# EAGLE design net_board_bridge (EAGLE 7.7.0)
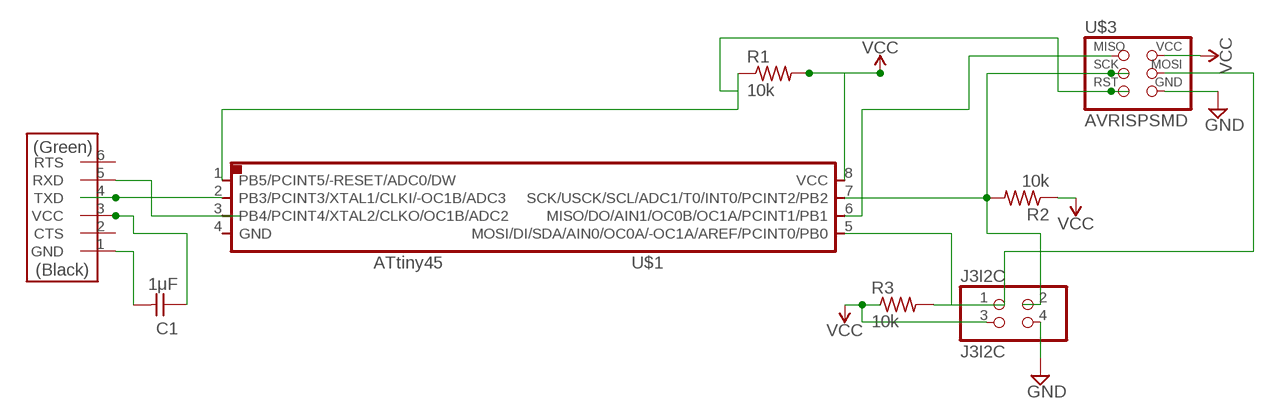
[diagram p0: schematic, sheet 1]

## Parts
C1  1μF  CAP-UNPOLARIZEDFAB  [C1206FAB]
J3I2C  J3I2C  PINHD-2X2-SMD  [2X02SMD]
R1  10k  RES-US1206FAB  [R1206FAB]
R2  10k  RES-US1206FAB  [R1206FAB]
R3  10k  RES-US1206FAB  [R1206FAB]
U$1  ATTINY45SI  [SOIC8]
U$2  FTDI-SMD-HEADER  [1X06SMD]
U$3  AVRISPSMD  [2X03SMD]

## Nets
GND: J3I2C.4 U$3.6(GND)
N$2: R1.1 U$1.1(PB5/PCINT5/-RESET/ADC0/DW) U$3.5(RST)
N$3: U$2.5(RXD)
N$4: R2.2 U$1.7(SCK/USCK/SCL/ADC1/T0/INT0/PCINT2/PB2) U$3.3(SCK)
N$6: R3.2 U$1.5(MOSI/DI/SDA/AIN0/OC0A/-OC1A/AREF/PCINT0/PB0) U$3.4(MOSI)
N$7: U$1.2(PB3/PCINT3/XTAL1/CLKI/-OC1B/ADC3) U$2.4(TXD)
N$8: C1.2 U$2.1(GND)
N$9: C1.1 U$2.3(VCC)
N$11: U$1.6(MISO/DO/AIN1/OC0B/OC1A/PCINT1/PB1) U$3.1(MISO)
VCC: J3I2C.3 R1.2 R2.1 R3.1 U$1.8(VCC) U$3.2(VCC)
Unconnected: J3I2C.1 J3I2C.2 U$1.3(PB4/PCINT4/XTAL2/CLKO/OC1B/ADC2) U$1.4(GND) U$2.2(CTS) U$2.6(RTS)

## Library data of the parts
C1 = fab:CAP-UNPOLARIZED
J3I2C = fab:PINHD-2X2-SMD
R1-R3 = fab:RES-US: Resistor (US Symbol)
U$1 = fab:ATTINY45
U$2 = fab:FTDI-SMD-HEADER
U$3 = fab:AVRISP

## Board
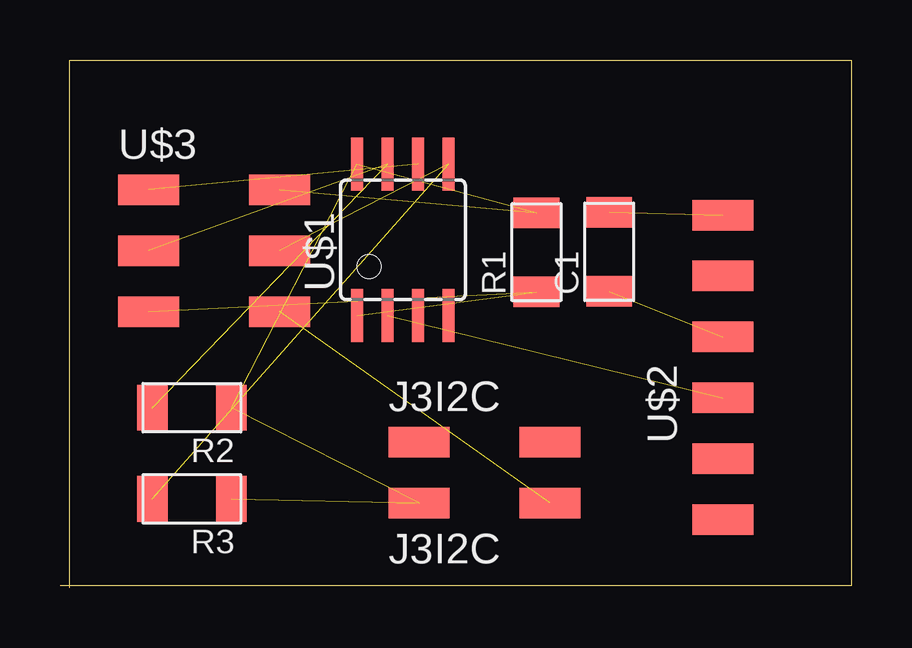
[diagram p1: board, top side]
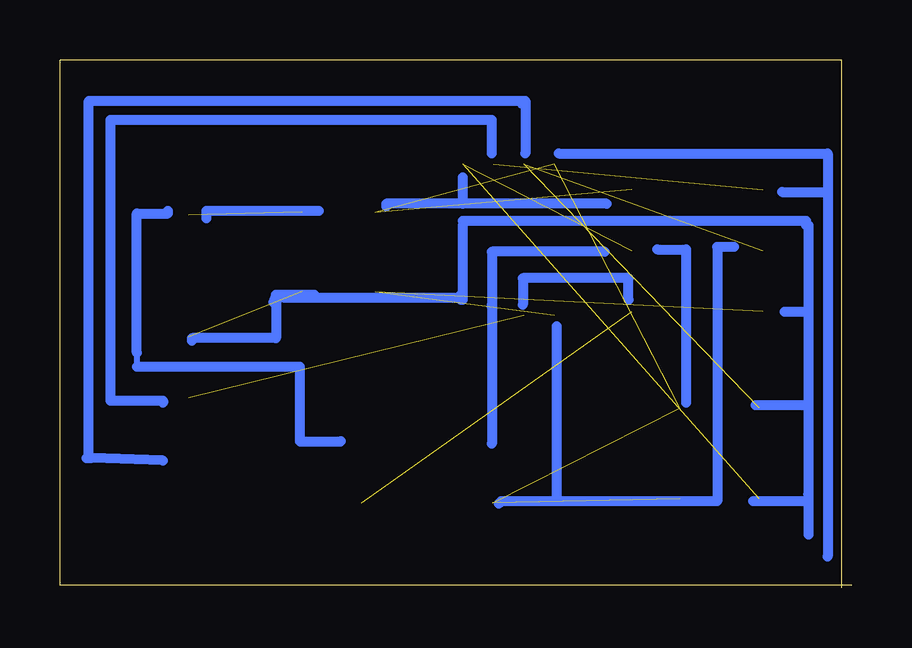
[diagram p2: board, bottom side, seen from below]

Size 33 x 22 mm. Coordinates in mm from the lower left corner, seen from the top.
Outline: 0,0.1 33,0.1 33,22 0.4,22 0.4,0
Copper layers (1*16): Top 0.035mm / dielectric 1.5mm / Bottom 0.035mm
Design rules "default": minimum track width 10mil, minimum drill 24mil, track to track 8mil, track to pad 8mil, pad to pad 8mil, via to via 8mil, smd to smd 8mil, copper to edge 40mil, drill to drill 8mil, minimum pad ring 10mil, minimum via ring 8mil, stop-mask expansion 4mil, vias tented up to drill 0mil, thermal gap 10mil

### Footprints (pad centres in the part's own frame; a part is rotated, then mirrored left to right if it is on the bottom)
C1206FAB = smd 1.27 x 1.905: 1 -1.651,0; 2 1.651,0
2X02SMD = smd 2.54 x 1.27: 1 -2.54,1.27; 2 2.92,1.27; 3 -2.54,-1.27; 4 2.92,-1.27
R1206FAB = smd 1.27 x 1.905: 1 -1.651,0; 2 1.651,0
SOIC8 = smd 0.5 x 2.2: 1 -1.905,-3.154; 2 -0.645,-3.154; 3 0.625,-3.154; 4 1.895,-3.154; 5 1.905,3.154; 6 0.635,3.154; 7 -0.635,3.154; 8 -1.905,3.154
1X06SMD = smd 2.54 x 1.27: 1 0,6.35; 2 0,3.81; 3 0,1.27; 4 0,-1.27; 5 0,-3.81; 6 0,-6.35
2X03SMD = smd 2.54 x 1.27: 1 -2.54,2.54; 2 2.92,2.54; 3 -2.54,0; 4 2.92,0; 5 -2.54,-2.54; 6 2.92,-2.54

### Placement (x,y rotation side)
C1  22.9,14 90 top
J3I2C  17.5,4.8 0 top
R1  19.86,13.98 90 top
R2  5.5,7.5 180 top
R3  5.5,3.7 180 top
U$1  14.3,14.5 0 top
U$2  27.64,9.18 0 top
U$3  6.23,14.05 0 top

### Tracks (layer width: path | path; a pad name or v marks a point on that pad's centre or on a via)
GND  (1 unrouted)
N$1
  Bottom 0.406: 22.2,15.7 26.9,15.7 26.9,15.4
N$2  (2 unrouted)
N$4  (2 unrouted)
N$5
  Bottom 0.406: 22.4,12.2 24,12.2 | 24.1,11.9 24,12.2 | 24,12.2 24,10.4 27.5,10.4 27.5,10.3
N$6  (2 unrouted)
N$7  (1 unrouted)
N$8  (1 unrouted)
N$9  (1 unrouted)
N$10
  Bottom 0.406: 23.7,12.1 16.3,12.1 16.3,12.2
N$11  (1 unrouted)
N$12
  Bottom 0.406: 7.5,3.6 12.3,3.6 | 12.3,3.6 14.6,3.6 14.7,3.5 | 12.3,10.9 12.3,3.6
N$13
  Bottom 0.406: 10.3,14 15,14 15,11.8 | 15,11.8 15,11.7 | 15,11.8 15,6
N$14
  Bottom 0.406: 16.3,12 16.2,12 16.2,15.1
N$15
  Bottom 0.406: 16.2,15.3 1.9,15.3
N$16
  Bottom 0.406: 2,3.6 4.1,3.6
N$17
  Bottom 0.406: 1.9,7.6 4,7.6
N$18
  Bottom 0.406: 1.9,15.1 1.8,15.1 1.8,3.7
N$19
  Bottom 0.406: 4.9,14.2 5.6,14.2 5.6,3.6 7.6,3.6
N$20
  Bottom 0.406: 8.1,14.1 6.9,14.1 6.9,7.7
N$21
  Bottom 0.406: 9.3,12 9.3,12.9 13.7,12.9 13.7,11.8
N$22
  Bottom 0.406: 10.2,16 16.2,16 | 16.2,16 19.4,16 19.4,15.9 | 16.2,16 16.2,17.1
N$23
  Bottom 0.406: 15,18.1 15,19.5 30.9,19.5 30.9,7.8 28.7,7.8 28.7,7.7
N$24
  Bottom 0.254: 13.7,20.2 13.8,20.1
  Bottom 0.406: 28.7,5.3 31.7,5.4 31.8,5.4 | 31.9,5.4 31.8,5.4 | 31.8,5.4 31.8,20.3 13.6,20.3 | 13.7,20.2 13.6,20.3 | 13.6,20.3 13.6,18.1
N$25
  Bottom 0.254: 1.9,3.9 1.8,3.9
  Bottom 0.406: 1.8,3.9 1.8,2.2
N$26
  Bottom 0.406: 12.2,18.1 1,18.1 1,16.5 | 2.9,16.5 1,16.5 | 1,16.5 1,1.3
N$27
  Bottom 0.406: 2.8,11.5 1.9,11.5
N$28
  Bottom 0.254: 29.8,9.8 29.8,9.2 | 21.6,6 23,6 23,6.1 | 21.3,6 21.3,6.1
  Bottom 0.406: 28.5,15.7 28.5,15.6 29.8,15.6 29.8,9.8 | 29.8,9.2 23,9.2 23,6.1 21.3,6.1
VCC  (5 unrouted)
